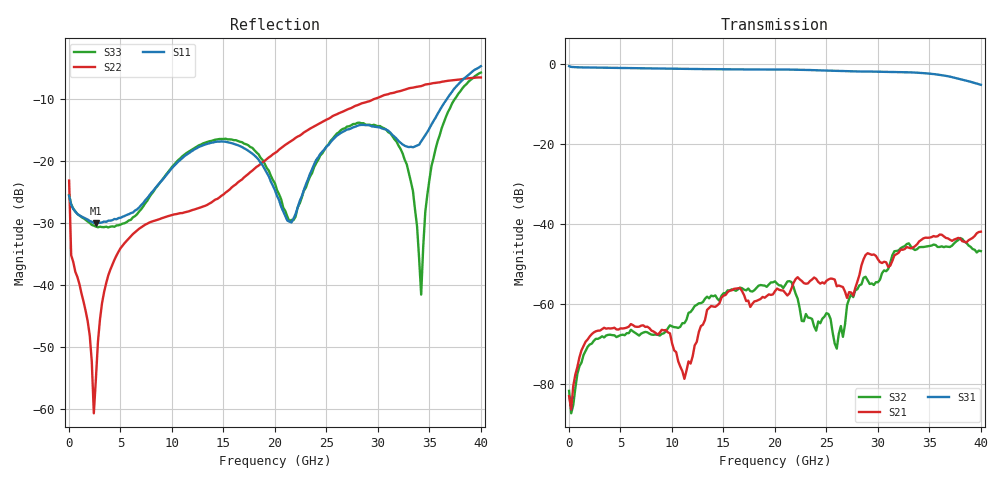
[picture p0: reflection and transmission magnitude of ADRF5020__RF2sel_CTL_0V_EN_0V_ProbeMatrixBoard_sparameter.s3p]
! Device:  ADRF5020
! Description: SOI MMIC SPDT Non-Reflective Switch
! Frequency:  0.1 -  30 GHz
! Ports:
! 	RFC	= Port 1
!	RF1	= Port 2
!	RF2	= Port 3
! Vdd:  +3.3 Volt
! Vss:  -2.5 Volt
! Control:  0/+3.3 Volt
! State:  RF2 Selected (Vctl= 0 V, Ven= 0 V)
! Data:  The device was measured using G-S-G Probes on a matrix board.
!  Data was collected using an calibrated 4 port network analyzer.
!  The reference plane is the package pins of ADRF5020 switch.
! Note:  Analog Devices supplies this data as a sample of measured data at the package pin
!  for this product.  Your particular data for this product may vary.
!  Data was taken at 25 degrees C.
!  Analog Devices reserves the right to change this data at anytime.
# GHZ S DB R 50.0
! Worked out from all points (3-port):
!   201 points, 10 MHz to 40.01 GHz, reference 50 ohm
!   strongest paths, dB at 10 MHz, 10.01 GHz, 20.01 GHz, 30.01 GHz, 40.01 GHz:
!     S31: -0.6, -1.2, -1.4, -2.0, -5.2
!     S21: -83.0, -69.8, -56.8, -48.8, -41.9
!     S32: -81.7, -65.6, -54.3, -54.6, -46.8
!   lowest |S11| = -30.0 dB at 2.61 GHz (marker M1), VSWR 1.07, Z = 52.1 - j2.43 ohm
!   |S11| at or under -10 dB: start of sweep to 36.69 GHz
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0.01  -25.59 -23.3  -78.75 124.3  -0.61 0.0
      -83.01 -19.3  -23.13 69.1  -77.19 -123.6
      -0.60 -0.0  -81.70 119.2  -25.45 -14.2
2.61  -29.98 -47.1  -66.98 46.5  -0.96 -30.4
      -66.81 44.6  -55.13 -69.2  -69.03 32.1
      -0.95 -30.4  -68.69 33.8  -30.55 -44.8
4.81  -29.17 -51.4  -66.23 32.5  -1.04 -55.5
      -66.38 32.1  -34.58 -73.2  -68.05 1.9
      -1.04 -55.5  -68.00 2.3  -30.34 -48.0
11.21  -19.21 -49.3  -78.61 -13.5  -1.27 -128.2
       -78.70 -8.9  -28.26 -71.2  -64.81 -99.4
       -1.27 -128.1  -64.78 -101.5  -18.95 -55.0
20.01  -24.70 -107.2  -56.84 100.9  -1.44 130.8
       -56.79 101.9  -18.68 -36.4  -54.38 68.8
       -1.44 130.9  -54.34 69.1  -23.61 -132.1
26.01  -15.91 -30.7  -55.60 75.7  -1.77 58.9
       -55.59 75.4  -12.46 -51.6  -71.64 -31.1
       -1.77 59.1  -71.16 -30.1  -15.57 -54.5
30.81  -14.92 -65.5  -49.57 85.4  -2.00 -0.2
       -49.59 85.0  -9.29 -71.8  -51.78 133.6
       -2.00 -0.0  -51.81 134.4  -14.94 -103.2
34.21  -16.82 -35.0  -44.03 82.3  -2.30 -46.2
       -44.01 82.7  -7.91 -88.5  -45.82 76.5
       -2.29 -46.0  -45.77 76.1  -41.51 -30.1
35.81  -12.38 -24.8  -43.05 62.2  -2.71 -69.5
       -43.08 62.1  -7.33 -98.0  -45.75 57.7
       -2.71 -69.3  -45.76 57.6  -16.78 6.7
40.01  -4.70 -59.2  -42.00 43.4  -5.24 -127.6
       -41.94 43.7  -6.52 -119.9  -46.97 19.7
       -5.25 -127.4  -46.79 20.6  -5.73 -45.4
